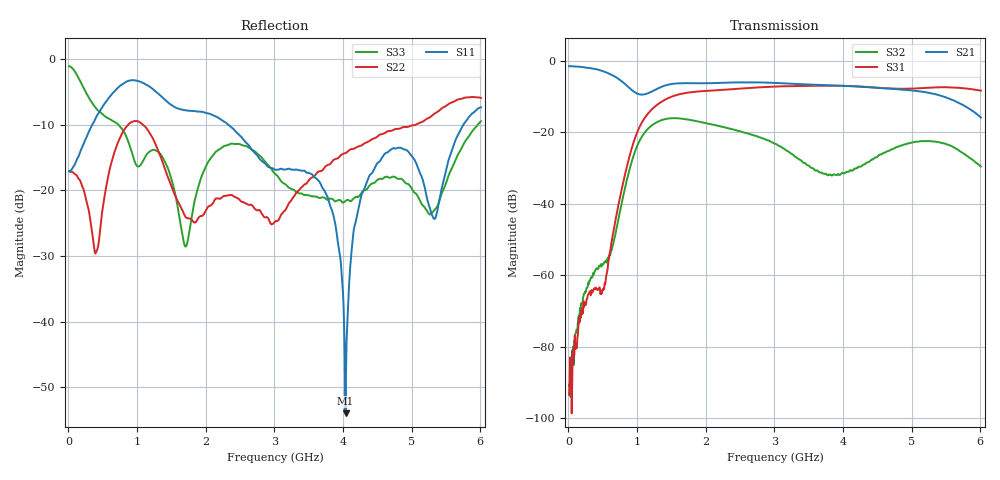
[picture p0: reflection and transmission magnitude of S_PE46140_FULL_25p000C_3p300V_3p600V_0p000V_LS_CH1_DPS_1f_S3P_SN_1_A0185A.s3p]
! Device ID: PE46140_FULL
! File Path: z:\PE46140\MajorStates\25p000C\3p300\LS_CH1_DPS_1f\PE46140_FULL_25p000C_3p300V_3p600V_0p000V_LS_CH1_DPS_1f_S3P_SN_1_A0185A.s3p
! Serial: 1
! Lot: A0185A
! Temp: 25.000C
! VDD: 3.300
! VSS: 0.000
! Control_Hi: 3.600
! Control_Lo: 0.000
! Logic State: LS_CH1_DPS_1f
! Port 1: RFIN
! Port 2: RFOUT1
! Port 3: RFOUT2
! ThroughPath:1-2
! IDD: 0.0003110599
! ISS: -1.196e-007
! Comment:
#  Hz  S  RI  R  50
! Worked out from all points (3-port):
!   801 points, 10 MHz to 6.01 GHz, reference 50 ohm
!   strongest paths, dB at 10 MHz, 1.51 GHz, 3.01 GHz, 4.51 GHz, 6.01 GHz:
!     S21: -1.5, -6.5, -6.2, -7.6, -15.9
!     S31: -93.4, -10.0, -7.2, -7.5, -8.3
!     S32: -91.0, -16.0, -23.2, -26.6, -29.5
!   lowest |S11| = -54.0 dB at 4.037 GHz (marker M1), VSWR 1.00, Z = 49.8 + j0.0277 ohm
!   |S11| at or under -10 dB: start of sweep to 346.1 MHz; 2.33 GHz to 5.753 GHz (3.424 GHz wide, 84.7 % of centre)
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1e7  0.1402 -0.0109  0.8418 -0.0244  -2.66e-05 -1.81e-05
     0.8419 -0.0243  0.14 -0.00677  -1.97e-05 -9.34e-06
     -2.3e-06 2.13e-05  2.2e-05 -1.77e-05  0.8808 -0.0832
3.55e8  -0.0161 -0.3218  0.4592 -0.6282  -0.000547 -0.000316
        0.4593 -0.6263  -0.00906 -0.0427  -0.000106 0.00102
        -0.000542 -0.000251  -0.000154 0.000978  -0.4043 -0.2107
1.165e9  -0.5853 0.224  -0.2047 -0.2879  -0.1835 -0.0274
         -0.2049 -0.2885  0.2134 -0.1872  -0.00283 0.1135
         -0.1838 -0.0278  -0.00294 0.1136  0.166 0.1009
1.705e9  -0.2852 0.2924  -0.4874 0.003  0.2595 0.2415
         -0.4874 0.003  0.0343 -0.0529  -0.0256 -0.1509
         0.2596 0.2419  -0.0255 -0.151  -0.0366 -0.00749
3.01e9  0.0182 0.1429  0.4092 0.2716  -0.3781 -0.2183
        0.4089 0.2725  -0.0577 -0.00127  0.0618 -0.031
        -0.3785 -0.2187  0.0618 -0.031  0.1249 -0.0492
3.7675e9  0.0254 0.0875  0.2752 -0.3639  -0.2303 0.3848
          0.2756 -0.3636  0.0772 0.1346  -0.0138 0.0212
          -0.2303 0.3848  -0.0138 0.0213  0.0824 -0.0208
4.0375e9  -0.00199 0.000278  0.0427 -0.4431  -0.00254 0.4457
          0.0432 -0.4432  0.1394 0.1326  0.0231 0.0148
          -0.00151 0.4452  0.0231 0.0147  0.0803 -0.0219
4.3825e9  -0.1035 -0.0765  -0.2529 -0.3445  0.2624 0.3388
          -0.253 -0.345  0.2158 0.0995  0.0144 -0.0358
          0.2627 0.3385  0.0143 -0.0361  0.1032 -0.0324
5.335e9  -0.0411 -0.0448  -0.1078 0.3255  0.3078 -0.2933
         -0.1088 0.3256  0.3831 -0.0377  0.0127 0.0731
         0.3081 -0.2926  0.0122 0.0729  0.0702 0.0111
6.01e9  -0.2976 -0.3104  0.153 0.0483  -0.1977 -0.3267
        0.1538 0.0484  0.247 -0.4432  0.0275 -0.0185
        -0.1988 -0.327  0.0278 -0.0184  0.3117 0.1274
